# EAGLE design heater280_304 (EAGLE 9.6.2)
DATABASE: Z:\Eigene Dateien\Anwendungsdaten\Eagle\partdb\exp.txt
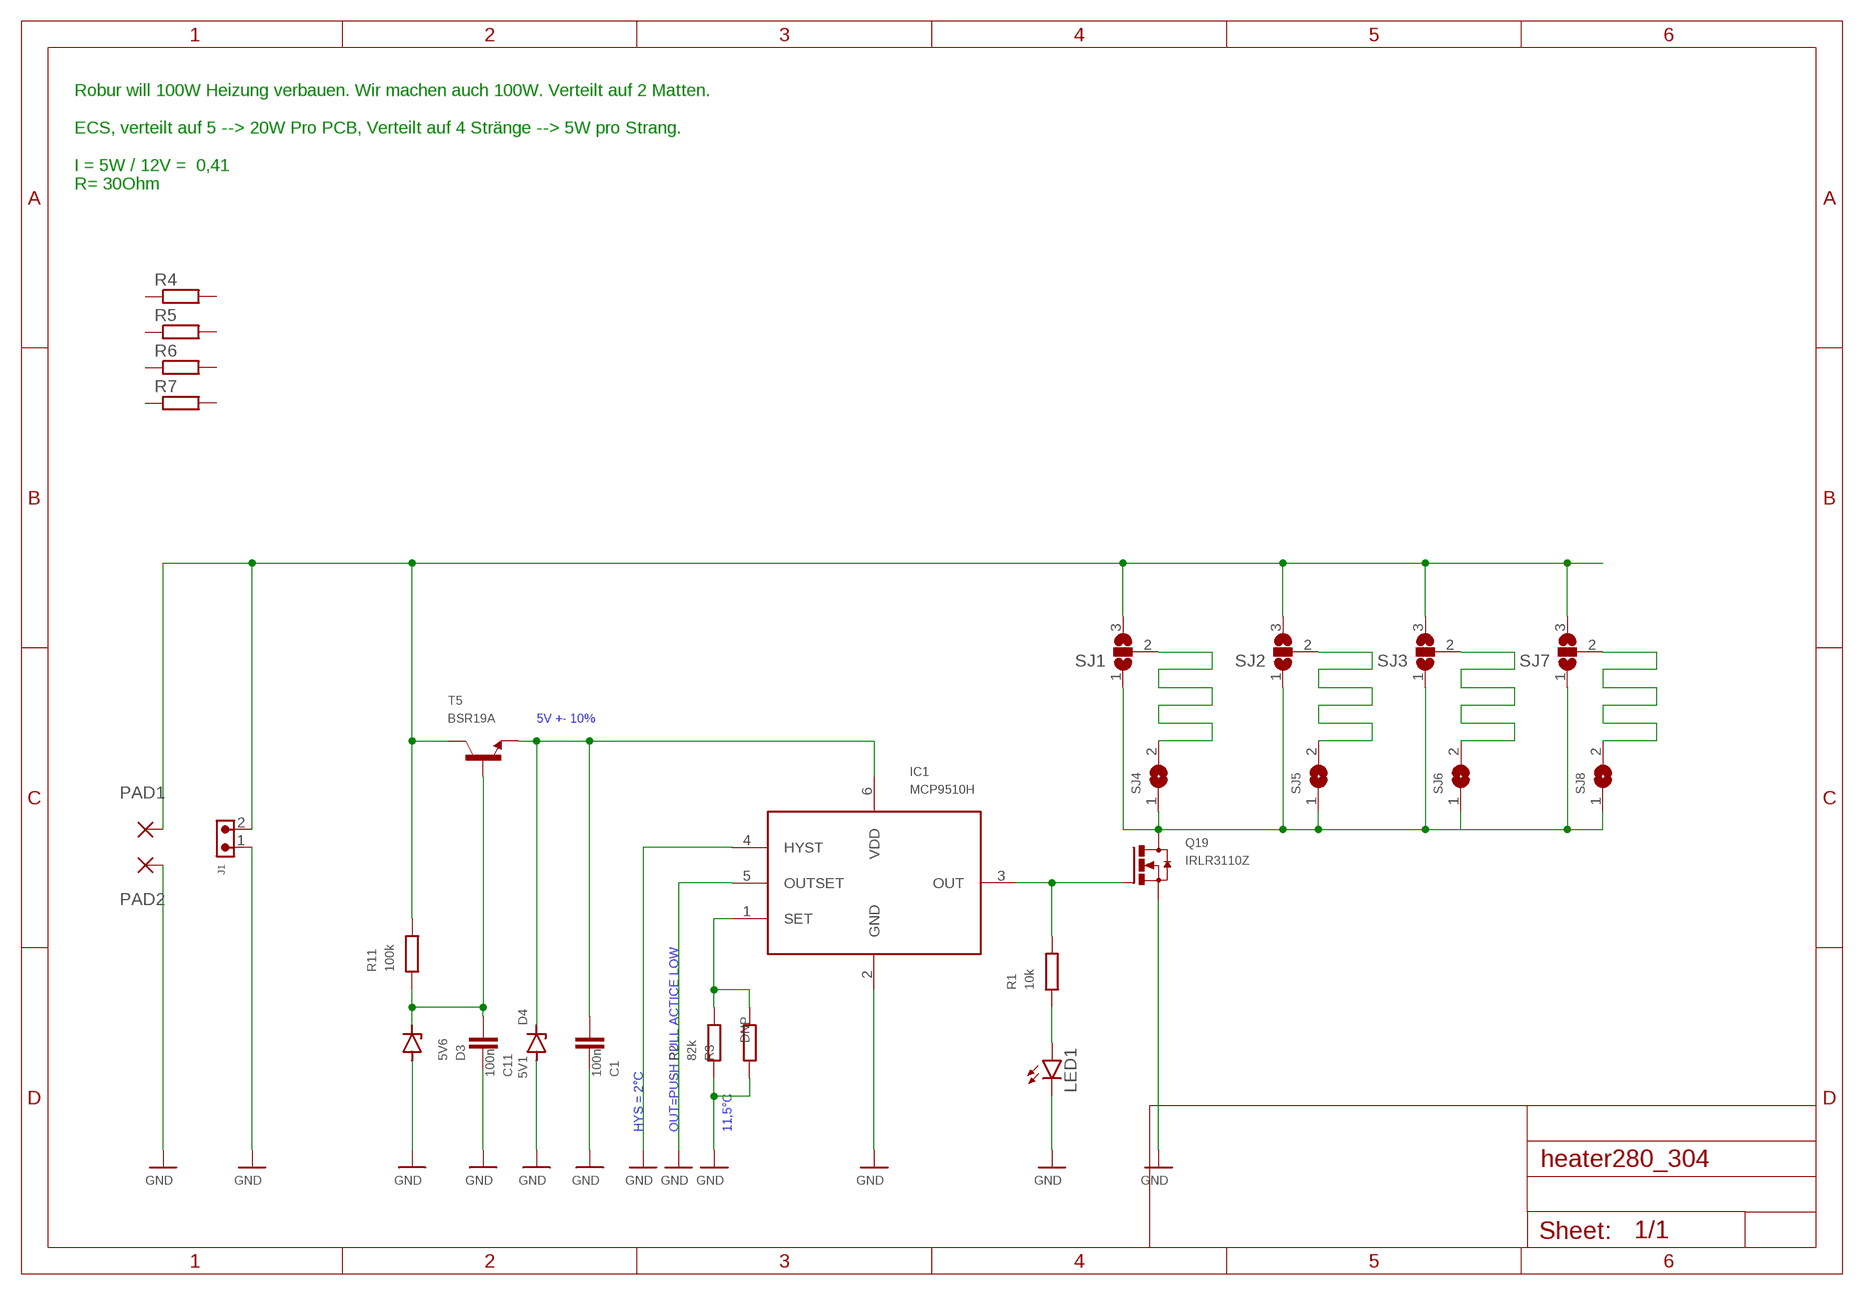
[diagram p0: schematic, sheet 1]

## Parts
C1  100n  C-EUC0603  [C0603]
C11  100n  C-EUC0603  [C0603]
D3  5V6  ZENER-DIODESOD80C  [SOD80C]
D4  5V1  ZENER-DIODESOD80C  [SOD80C]
IC1  MCP9510H  MCP9509  [SOT23-6]
J1  691322110002  [691322110002]
LED1  LEDSML0603  [SML0603]
PAD1  3,81/1,4  [3,81/1,4]
PAD2  3,81/1,4  [3,81/1,4]
Q19  IRLR3110Z  IRFR2607  [D-PACK]
R1  10k  R-EU_R0603  [R0603]
R2  82k  R-EU_R0603  [R0603]
R3  R-EU_R0603  [R0603]
R4  R-EU_R1206  [R1206]
R5  R-EU_R1206  [R1206]
R6  R-EU_R1206  [R1206]
R7  R-EU_R1206  [R1206]
R11  100k  R-EU_R0603  [R0603]
SJ1  SJ2W  [SJ_2]
SJ2  SJ2W  [SJ_2]
SJ3  SJ2W  [SJ_2]
SJ4  SJ  [SJ]
SJ5  SJ  [SJ]
SJ6  SJ  [SJ]
SJ7  SJ2W  [SJ_2]
SJ8  SJ  [SJ]
T5  BSR19A  MMBT2222ALT1-NPN-SOT23-BEC  [SOT23-BEC]

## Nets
+UB: J1.2 PAD1.1(P) R11.2 SJ1.3 SJ2.3 SJ3.3 SJ7.3 T5.C
GND: C1.2 C11.2 D3.A D4.A IC1.2(GND) IC1.4(HYST) IC1.5(OUTSET) J1.1 LED1.C PAD2.1(P) Q19.3(S) R2.1 R3.1
N$1: IC1.3(OUT) Q19.1(G) R1.2
N$2: SJ1.2 SJ4.2
N$3: C11.1 D3.C R11.1 T5.B
N$4: IC1.1(SET) R2.2 R3.2
N$5: C1.1 D4.C IC1.6(VDD) T5.E
N$6: LED1.A R1.1
N$7: SJ2.2 SJ5.2
N$8: SJ3.2 SJ6.2
N$9: SJ7.2 SJ8.2
N$11: Q19.4(D) SJ1.1 SJ2.1 SJ3.1 SJ4.1 SJ5.1 SJ6.1 SJ7.1 SJ8.1
Unconnected: R4.1 R4.2 R5.1 R5.2 R6.1 R6.2 R7.1 R7.2

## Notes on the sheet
- Robur will 100W Heizung verbauen. Wir machen auch 100W. Verteilt auf 2 Matten.
  
  ECS, verteilt auf 5 --> 20W Pro PCB, Verteilt auf 4 Stränge --> 5W pro Strang.
  
  I = 5W / 12V =  0,41
  R= 30Ohm
- 5V +- 10%
- HYS = 2°C | OUT=PUSH PULL ACTICE LOW | 11,5°C

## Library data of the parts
C1 C11 = rcl:C-EU: CAPACITOR, European symbol; PARTNO: C067; SPICEPREFIX: C
D3 = diode:ZENER-DIODE: Z-Diode; PARTNO: D013
D4 = diode:ZENER-DIODE: Z-Diode; PARTNO: D012
IC1 = mcp9509:MCP9509; PARTNO: IC333
J1 = Wurth_Connectors_WR-TBL Pluggable Connector:691322110002: WR-TBL Serie 3221 - 3.50 mm Horizontal PCB Header; DATASHEET-URL: https://www.we-online.com/catalog/datasheet/691322110002.pdf; IR-UL: 10A; IR-VDE: 10.5A; MOUNT: THT; PART-NUMBER: 691322110002; PARTNO: CON212; PINS: 2; PITCH: 3.5mm; TYPE: Horizontal; WORKING-VOLTAGE-UL: 300V (AC); WORKING-VOLTAGE-VDE: 300V (AC)
LED1 = led:LED: LED; PARTNO: D078
PAD1 PAD2 = wirepad:3,81/1,4: THROUGH-HOLE PAD
Q19 = IRFR2607:IRFR2607; PARTNO: T086
R1 = rcl:R-EU_: RESISTOR, European symbol; PARTNO: R221; SPICEPREFIX: R
R2 = rcl:R-EU_: RESISTOR, European symbol; PARTNO: R243; SPICEPREFIX: R
R3 = rcl:R-EU_: RESISTOR, European symbol; DNP: T; PARTNO: R245; SPICEPREFIX: R
R4-R7 = rcl:R-EU_: RESISTOR, European symbol; PARTNO: R493; SPICEPREFIX: R
R11 = rcl:R-EU_: RESISTOR, European symbol; PARTNO: R245; SPICEPREFIX: R
SJ1-SJ3 SJ7 = jumper:SJ2W: SMD solder JUMPER
SJ4-SJ6 SJ8 = jumper:SJ: SMD solder JUMPER
T5 = transistor-neu-to92:*-NPN-: NPN Transistror; PARTNO: T056

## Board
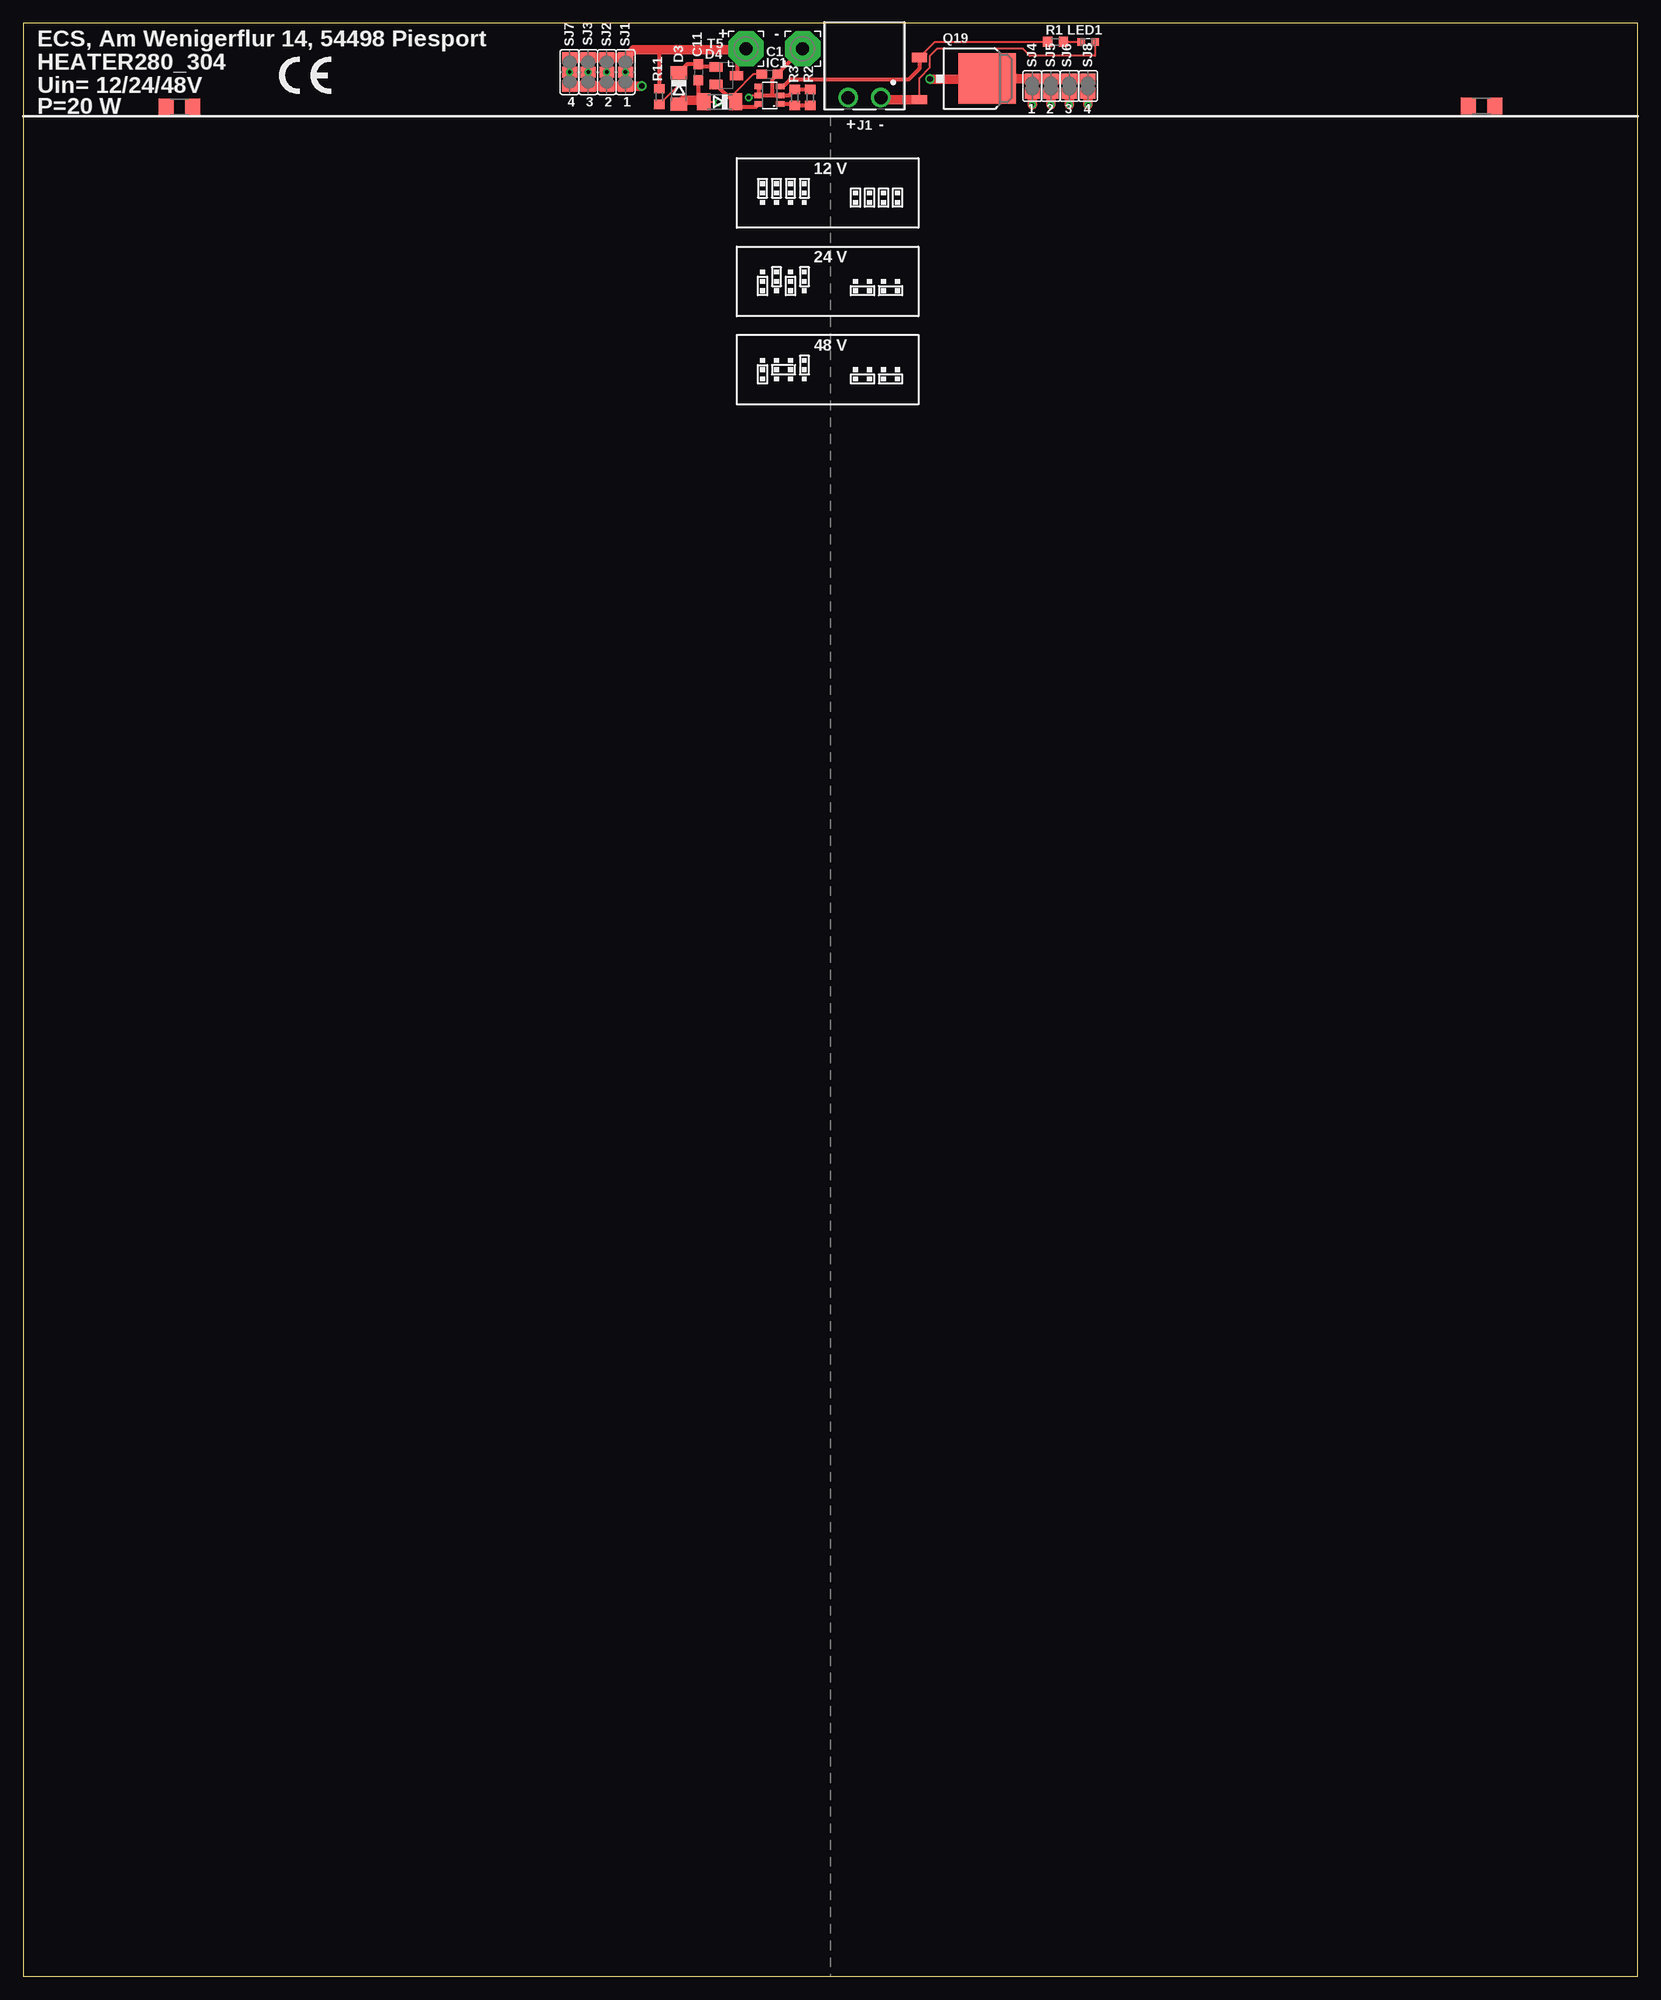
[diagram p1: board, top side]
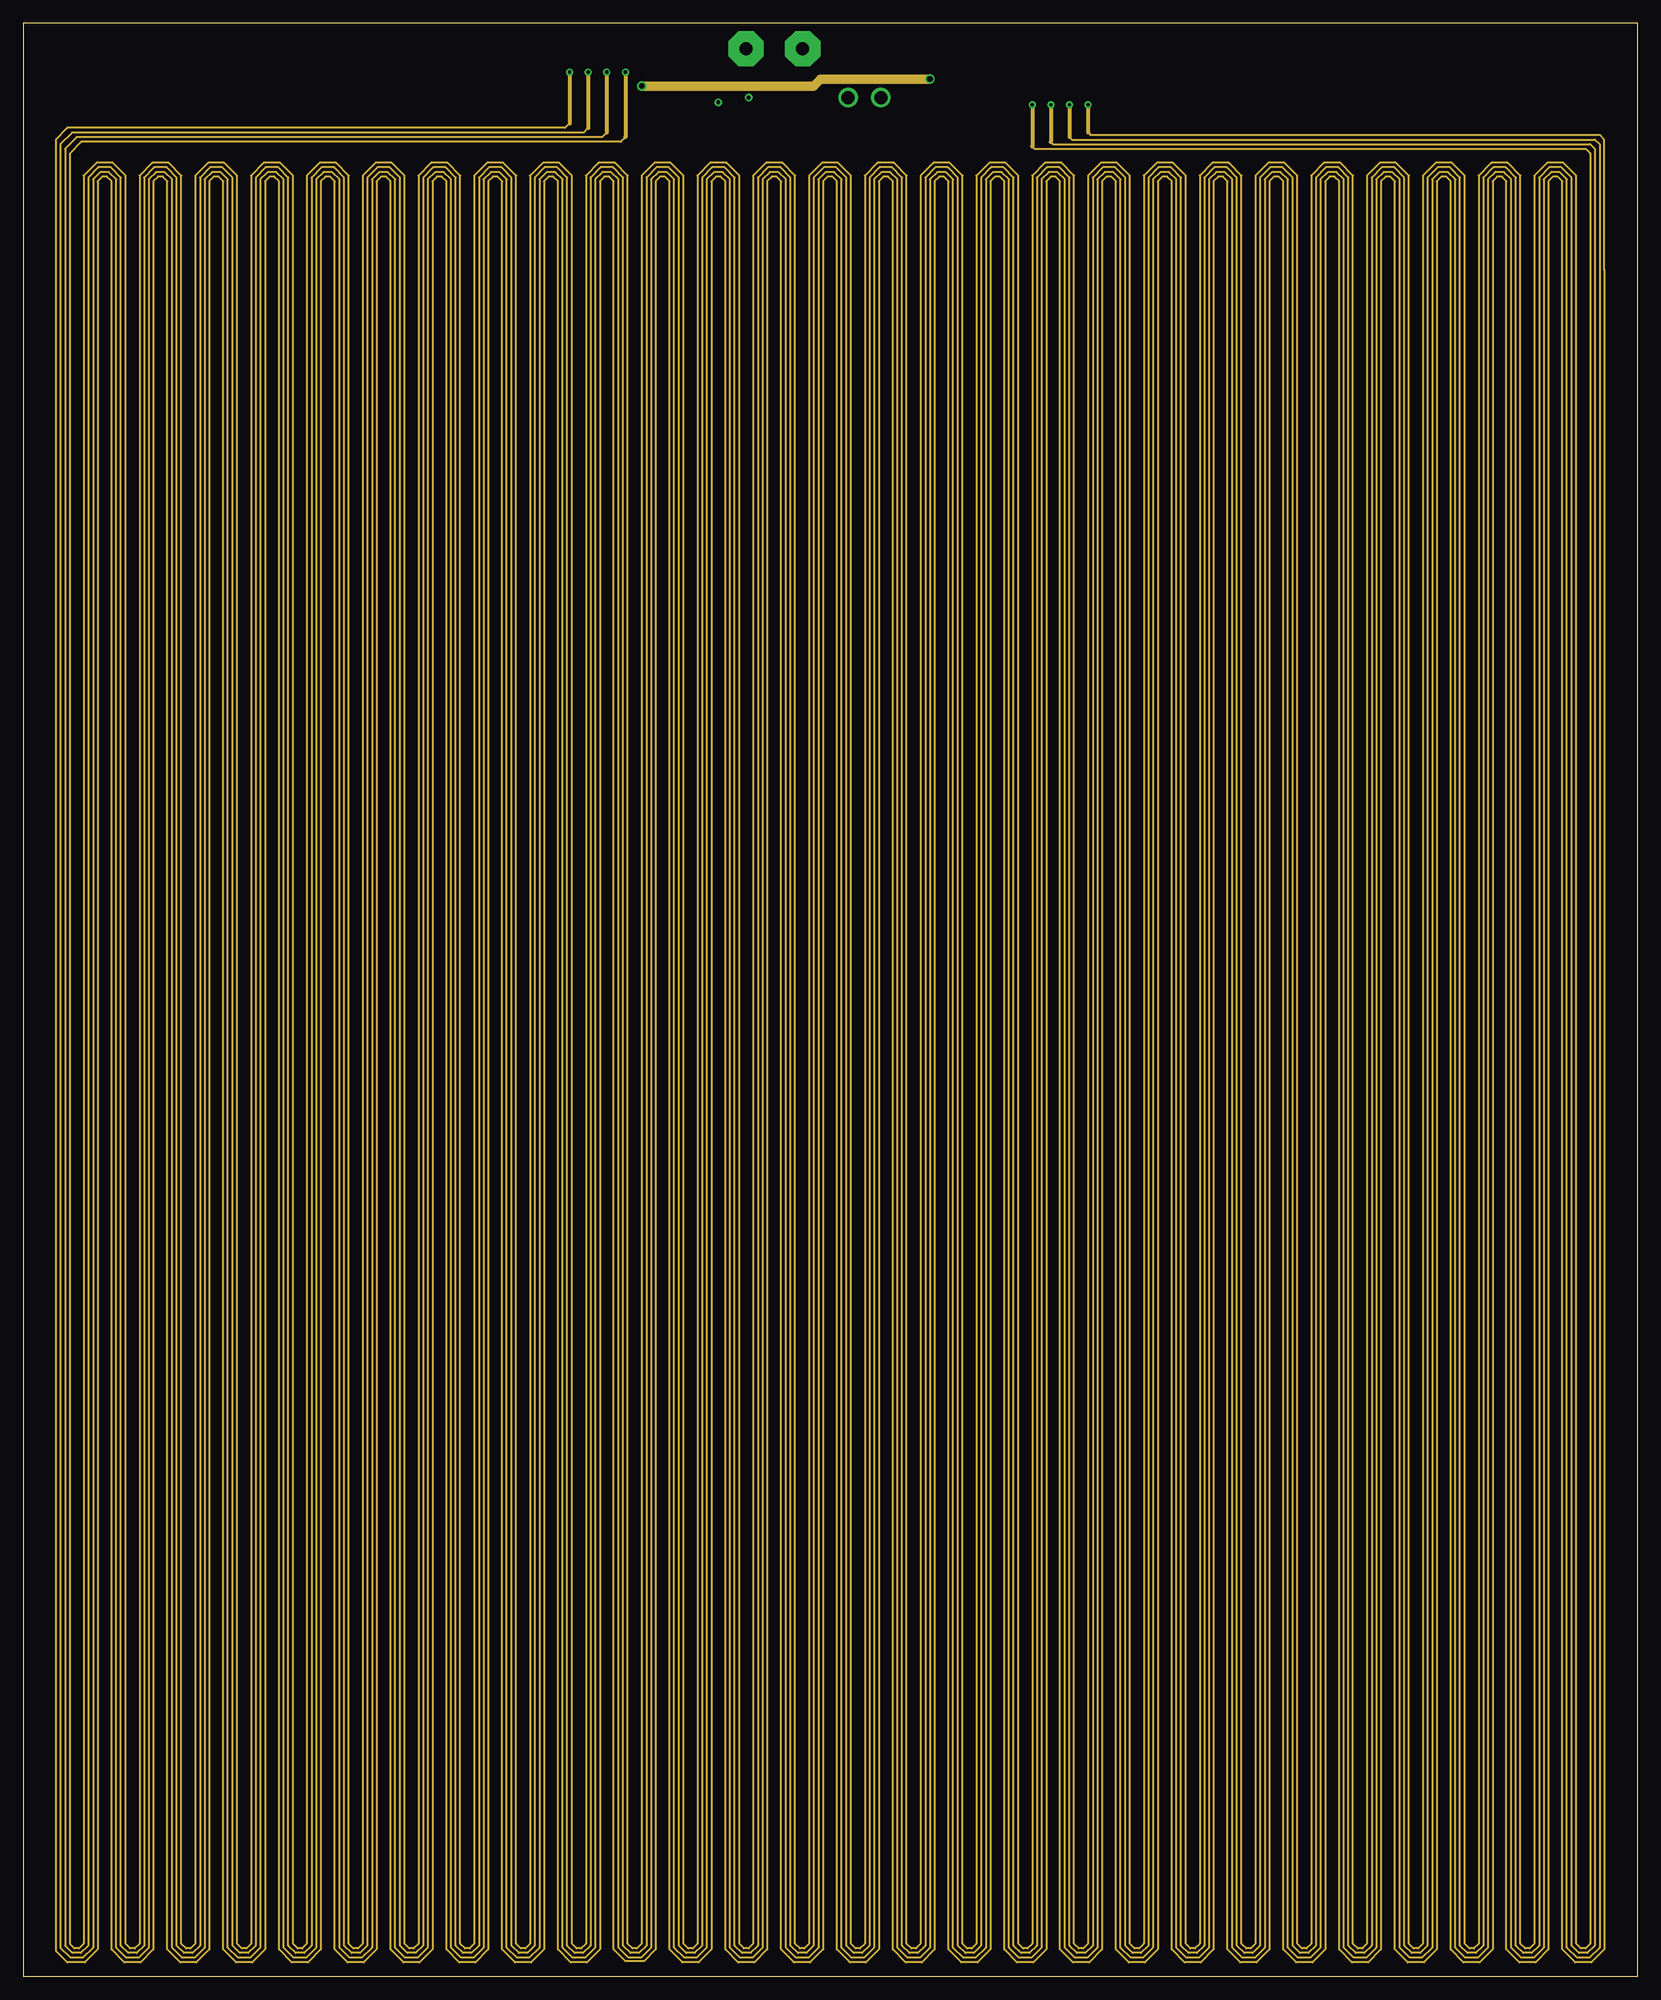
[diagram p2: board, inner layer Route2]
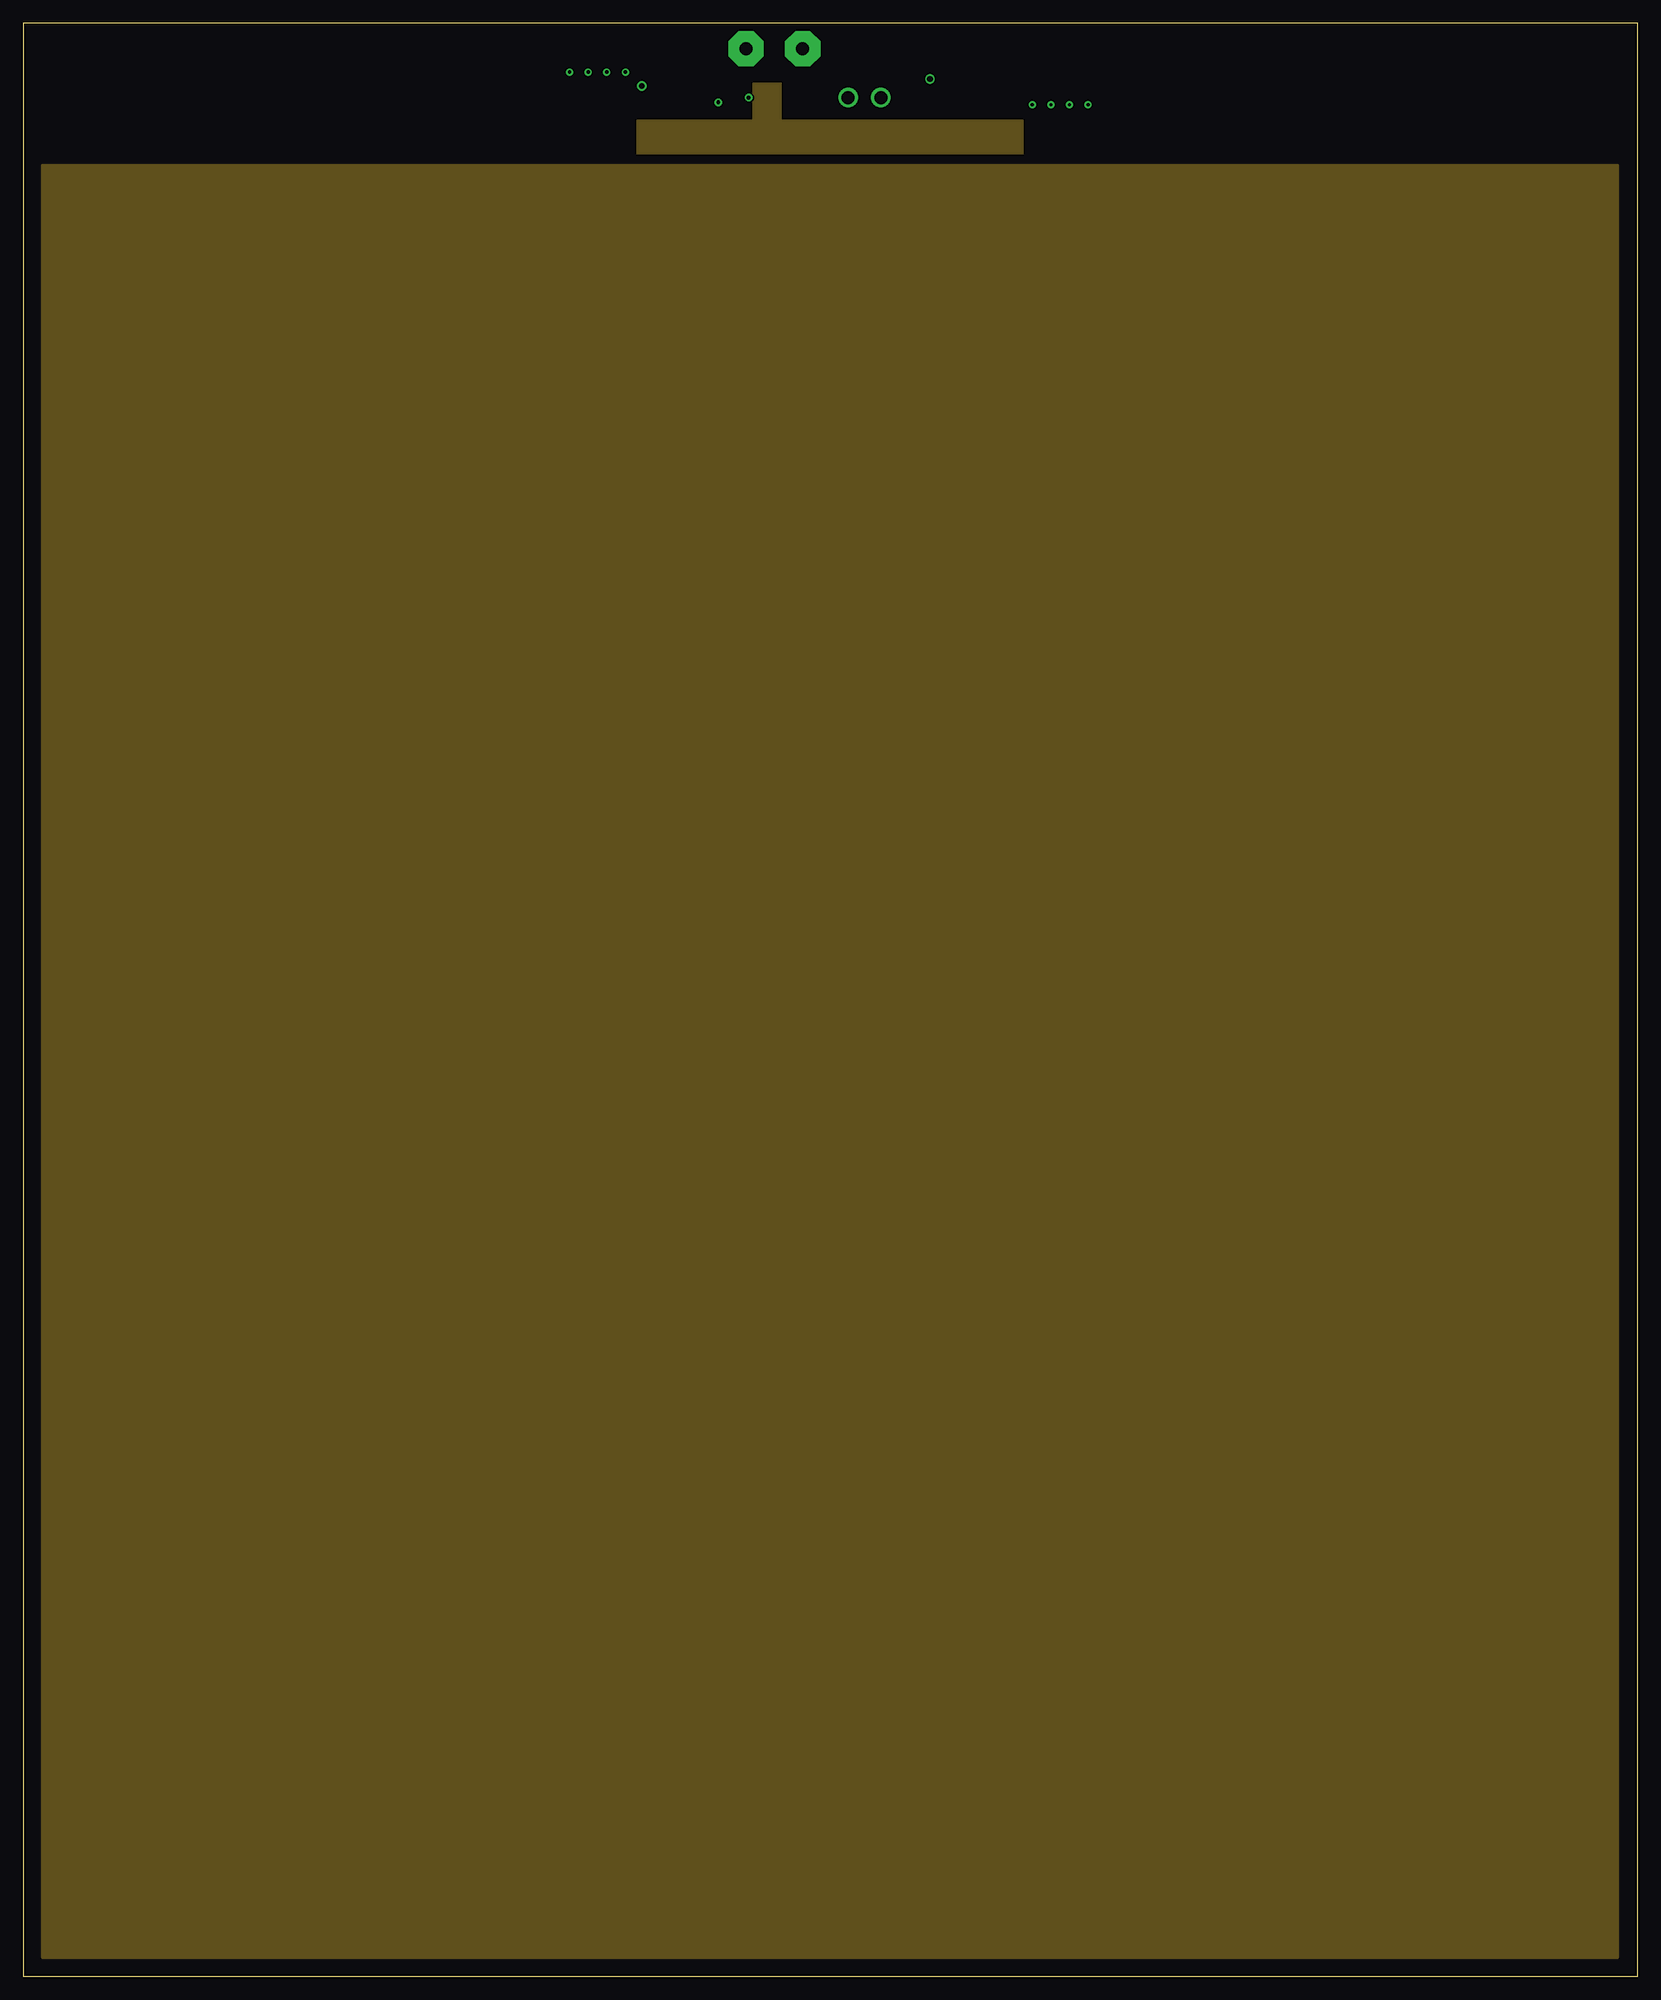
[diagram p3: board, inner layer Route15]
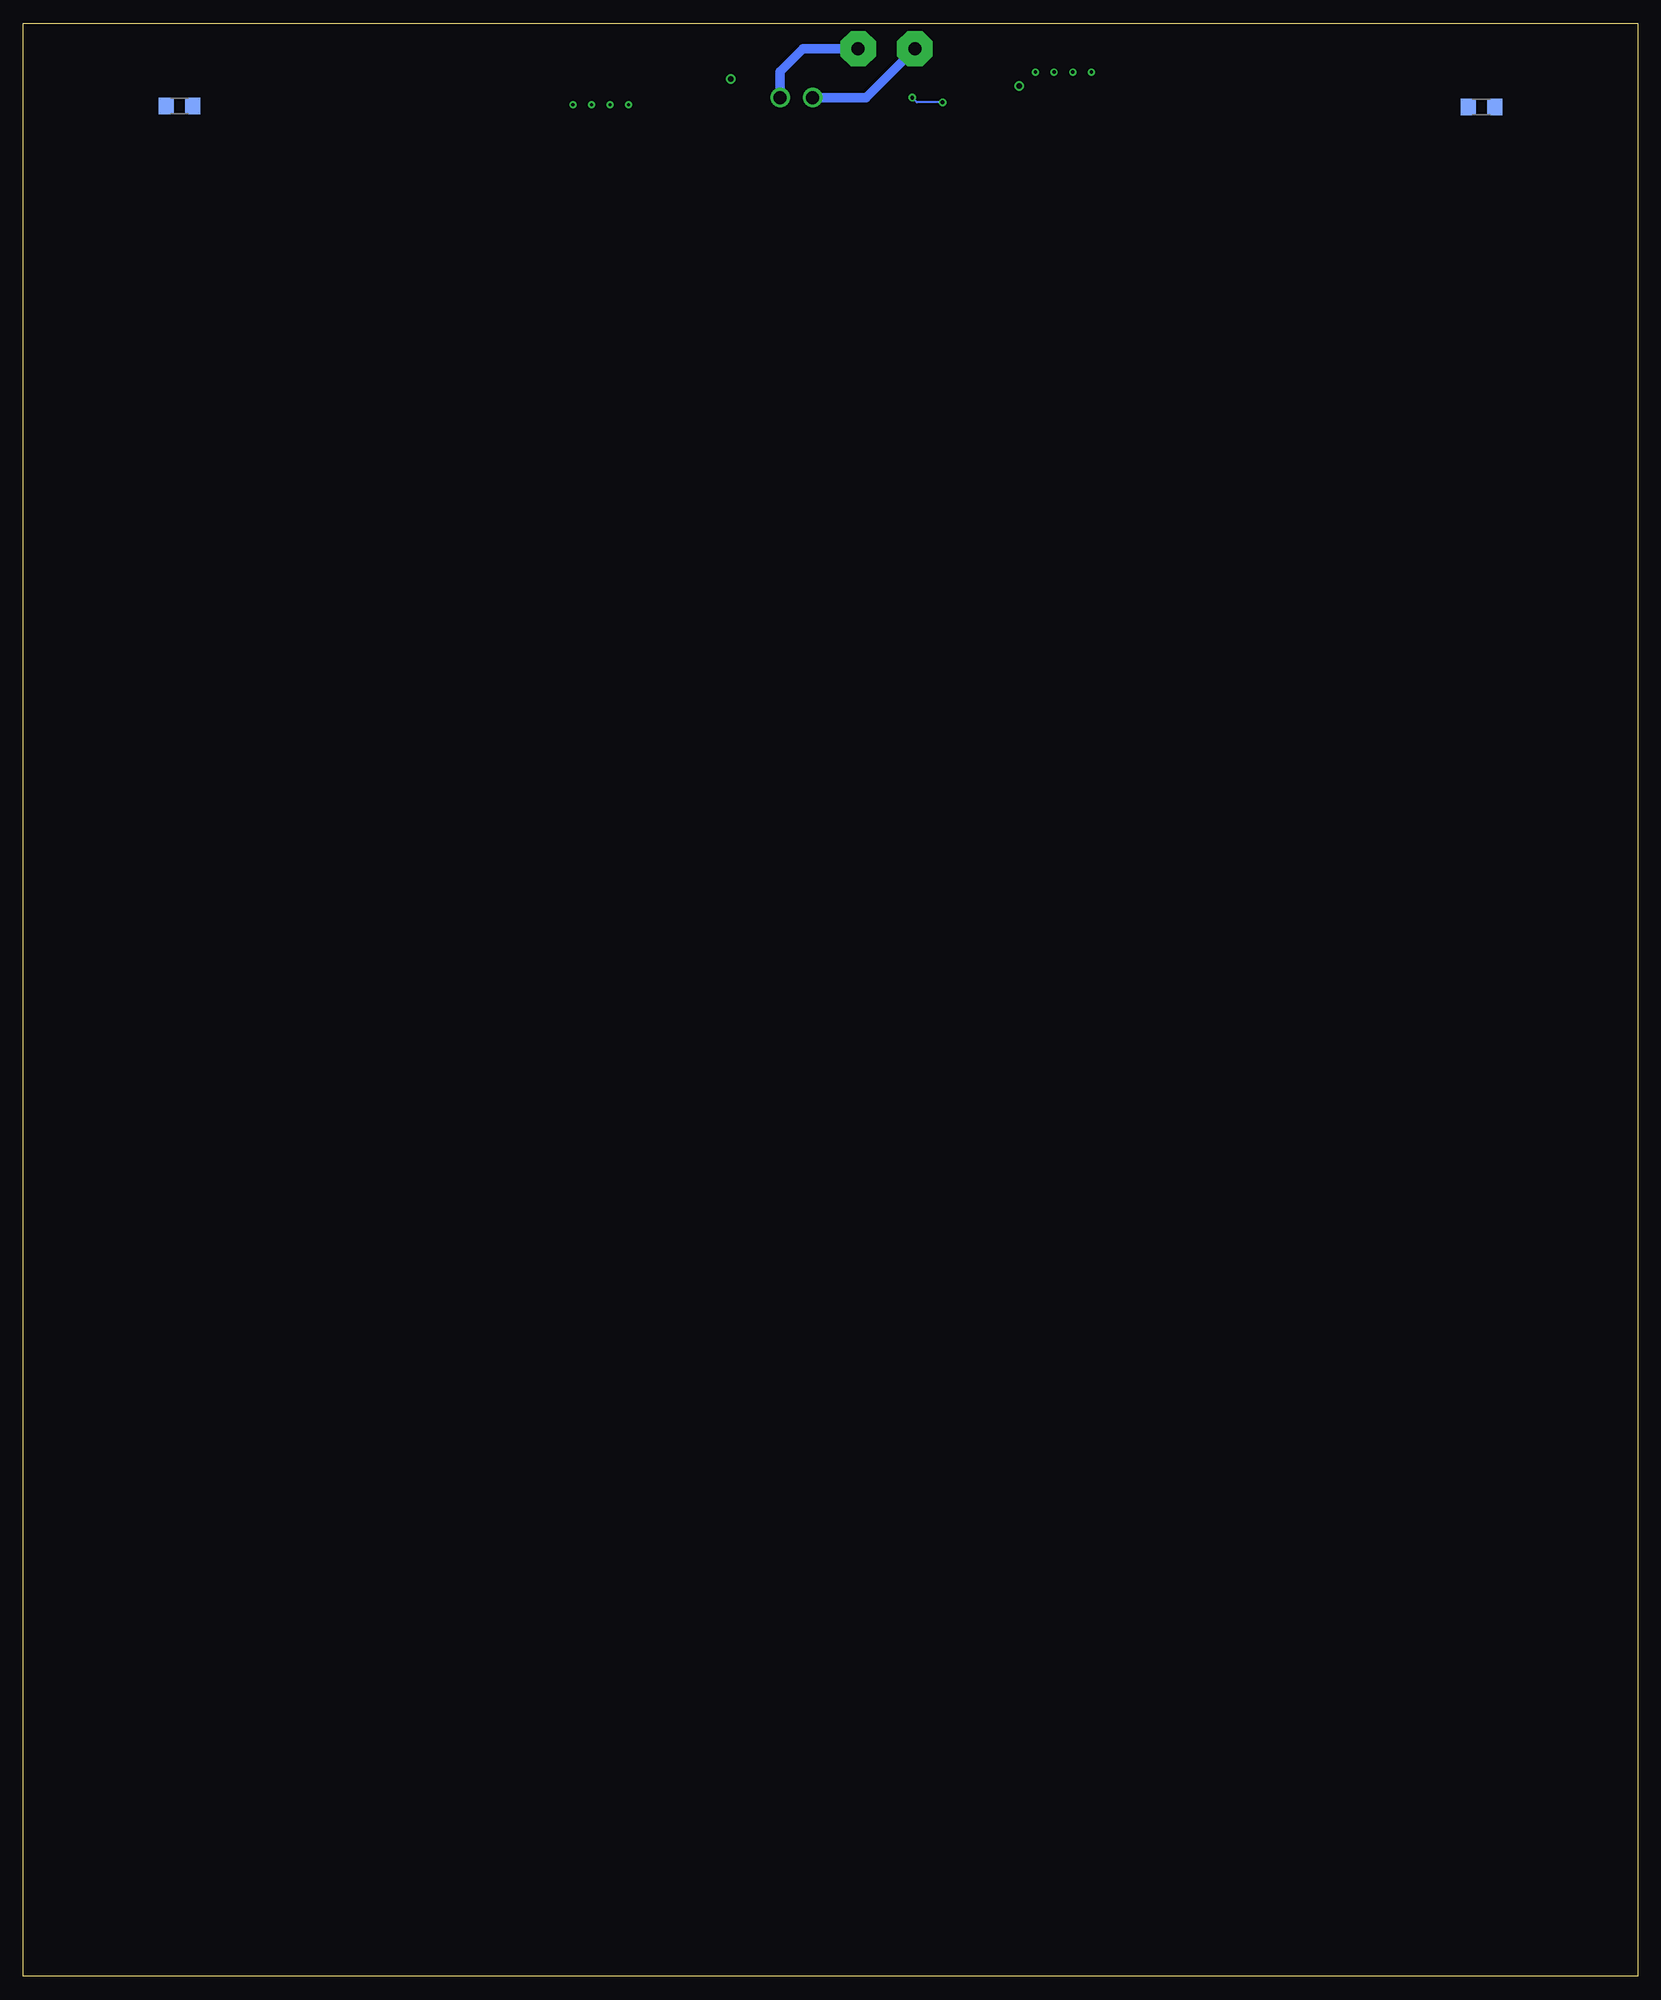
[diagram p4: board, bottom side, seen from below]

Size 173.6 x 210 mm. Coordinates in mm from the lower left corner, seen from the top.
Outline: 0,0 173.6,0 173.6,210 0,210 0,0
Copper layers (1+2*15+16): Top 0.035mm / dielectric 1.5mm / Route2 0.035mm / dielectric 0.15mm / Route15 0.035mm / dielectric 0.2mm / Bottom 0.035mm
Design rules "default *": minimum track width 6mil, minimum drill 0.35mm, track to track 6mil, track to pad 6mil, pad to pad 6mil, via to via 6mil, smd to smd 6mil, copper to edge 40mil, drill to drill 6mil, minimum pad ring 10mil, minimum via ring 8mil, stop-mask expansion 4mil, vias tented up to drill 0mil, thermal gap 10mil

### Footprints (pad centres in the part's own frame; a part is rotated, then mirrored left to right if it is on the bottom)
C0603 = smd 1.1 x 1: 1 -0.85,0; 2 0.85,0
SOD80C = smd 1.4 x 1.8: A 1.7,0; C -1.7,0
SOT23-6 = smd 0.6 x 0.9: 1 -0.95,-1.15; 2 0,-1.15; 3 0.95,-1.15; 4 0.95,1.15; 5 0,1.15; 6 -0.95,1.15
691322110002 = drill 1.4: 1 -1.75,0; 2 1.75,0
SML0603 = smd 0.8 x 0.8: A 0.75,0; C -0.75,0
3,81/1,4 = drill 1.397 pad 3.81 octagon: 1 0,0
D-PACK = smd 1 x 1.6: 1 -2.28,-4.8; 3 2.28,-4.8 | smd 5.4 x 6.2: 4 0,2.5
R0603 = smd 1 x 1.1: 1 -0.85,0; 2 0.85,0
R1206 = smd 1.6 x 1.803: 1 -1.422,0; 2 1.422,0
SJ_2 = smd 1.168 x 1.6: 1 -1.524,0; 2 0,0; 3 1.524,0
SJ = smd 1.168 x 1.6: 1 -0.762,0; 2 0.762,0
SOT23-BEC = smd 1 x 1.4: B -0.95,-1.1; C 0,1.1; E 0.95,-1.1

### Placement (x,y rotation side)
C1  80.27,204.52 0 top
C11  72.6,204.73 270 top
D3  70.5,203 270 top
D4  74.88,201.55 180 top
IC1  80.25,202.25 90 top
J1  90.46,202.01 180 top
LED1  114.5,208 180 top
PAD1  77.72,207.26 0 top
PAD2  83.82,207.26 0 top
Q19  101.16,204.05 270 top
R1  111,208 180 top
R2  84.64,202.02 270 top
R3  82.97,202.02 270 top
R4  16.8,201 180 top
R5  16.8,201 0 bottom
R6  156.8,201.1 0 top
R7  156.8,201.1 0 bottom
R11  68.4,202.12 90 top
SJ1  64.75,204.75 90 top
SJ2  62.75,204.75 90 top
SJ3  60.75,204.75 90 top
SJ4  108.5,203.25 270 top
SJ5  110.5,203.25 270 top
SJ6  112.5,203.25 270 top
SJ7  58.75,204.75 90 top
SJ8  114.5,203.25 270 top
T5  75.61,204.36 270 top
U$1  [CE-4MM]  27.5,202.38 0 top

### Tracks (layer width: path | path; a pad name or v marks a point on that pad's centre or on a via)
+UB
  Top 0.406: T5.C 76.75,204.4 76.75,206.29 77.61,207.15 PAD1.1 | R11.2 68.4,207.04 68.5,207.15
  Top 1.016: SJ7.3 SJ3.3 SJ2.3 SJ1.3 65.62,207.15 68.5,207.15 77.61,207.15
  Bottom 1.016: PAD1.1 82.97,202.01 J1.2
GND  (via drill 0.4)
  Top 0.2: LED1.C 115.25,206.5 108.25,206.5 107.5,207.25 98.25,207.25 97.5,206.5 97.5,205.25 96.36,204.11 Q19.3 | D4.A 74.7,201.55 v74.75,201.5 | v78,202 78.25,202.25 IC1.5
  Top 0.406: D4.A 72.6,202.13 C11.2 | 80.56,202.25 IC1.2 82.35,202.25 R3.1 R2.1 | 80.56,202.25 80.56,203.96 C1.2 81.12,204.56 PAD2.1 | IC1.4 IC1.5 80.56,202.25
  Top 1.016: D3.A 70.95,201.75 72.98,201.75 D4.A | Q19.3 92.45,201.77 J1.1
  Bottom 0.2: v74.75,201.5 77.5,201.5 v78,202
  Bottom 1.016: J1.1 92.21,204.79 89.74,207.26 PAD2.1
N$1
  Top 0.2: Q19.1 98.03,208 R1.2
  Top 0.406: IC1.3 81.7,203.2 82.5,204 95.25,204 96.36,205.11 Q19.1
N$2  (via drill 0.35, 0.35 pad 0.21)
  Top 1.016: SJ4.2 v108.5,201.25
  Route2 0.2: 108.5,196.75 108.75,196.5 168,196.5 168.5,196 168.5,3.5 168,3 167.5,3 167,3.5 167,193.62 165.62,195 163.88,195 162.5,193.62 162.5,3.5 162,3 161.5,3 161,3.5 161,193.62 159.62,195 157.88,195 156.5,193.62 156.5,3.5 156,3 155.5,3 155,3.5 155,193.62 153.62,195 151.88,195 150.5,193.62 150.5,3.5 150,3 149.5,3 149,3.5 149,193.62 147.62,195 145.88,195 144.5,193.62 144.5,3.5 144,3 143.5,3 143,3.5 143,193.62 141.62,195 139.88,195 138.5,193.62 138.5,3.5 138,3 137.5,3 137,3.5 137,193.62 135.62,195 133.88,195 132.5,193.62 132.5,3.5 132,3 131.5,3 131,3.5 131,193.62 129.62,195 127.88,195 126.5,193.62 126.5,3.5 126,3 125.5,3 125,3.5 125,193.62 123.62,195 121.88,195 120.5,193.62 120.5,3.5 120,3 119.5,3 119,3.5 119,193.62 117.62,195 115.88,195 114.5,193.62 114.5,3.5 114,3 113.5,3 113,3.5 113,193.62 111.62,195 109.88,195 108.5,193.62 108.5,3.5 108,3 107.5,3 107,3.5 107,193.62 105.62,195 103.88,195 102.5,193.62 102.5,3.5 102,3 101.5,3 101,3.5 101,193.62 99.62,195 97.88,195 96.5,193.62 96.5,3.5 96,3 95.5,3 95,3.5 95,193.62 93.62,195 91.88,195 90.5,193.62 90.5,3.5 90,3 89.5,3 89,3.5 89,193.62 87.62,195 85.88,195 84.5,193.62 84.5,3.5 84,3 83.5,3 83,3.5 83,193.62 81.62,195 79.88,195 78.5,193.62 78.5,3.5 78,3 77.5,3 77,3.5 77,193.62 75.62,195 73.88,195 72.5,193.62 72.5,3.5 72,3 71.5,3 71,3.5 71,193.62 69.62,195 67.88,195 66.5,193.62 66.5,3.5 66,3 65.5,3 65,3.5 65,193.62 63.62,195 61.88,195 60.5,193.62 60.5,3.5 60,3 59.5,3 59,3.5 59,193.62 57.62,195 55.88,195 54.5,193.62 54.5,3.5 54,3 53.5,3 53,3.5 53,193.62 51.62,195 49.88,195 48.5,193.62 48.5,3.5 48,3 47.5,3 47,3.5 47,193.62 45.62,195 43.88,195 42.5,193.62 42.5,3.5 42,3 41.5,3 41,3.5 41,193.62 39.62,195 37.88,195 36.5,193.62 36.5,3.5 36,3 35.5,3 35,3.5 35,193.62 33.62,195 31.88,195 30.5,193.62 30.5,3.5 30,3 29.5,3 29,3.5 29,193.62 27.62,195 25.88,195 24.5,193.62 24.5,3.5 24,3 23.5,3 23,3.5 23,193.62 21.62,195 19.88,195 18.5,193.62 18.5,3.5 18,3 17.5,3 17,3.5 17,193.62 15.62,195 13.88,195 12.5,193.62 12.5,3.5 12,3 11.5,3 11,3.5 11,193.62 9.62,195 7.88,195 6.5,193.62 6.5,3.5 6,3 5.5,3 5,3.5 5,196 6.26,197.25 64.25,197.25 64.75,197.75
  Route2 0.406: v108.5,201.25 108.5,196.75 | SJ1.2 64.75,197.75
  other vias: 64.75,204.75
N$3
  Top 0.2: R11.1 70.5,203.37 D3.C
  Top 0.406: D3.C 71.38,205.58 C11.1 72.87,205.31 T5.B
N$4
  Top 0.406: IC1.1 82.97,201.3 R3.2 R2.2
N$5
  Top 0.2: C1.1 79.4,204.5 78.5,204.5 76.58,202.58 D4.C
  Top 0.406: T5.E 76.37,201.55 D4.C 76.83,201.3 76.95,201.3 77.25,201 78.77,201 IC1.6
N$6
  Top 0.2: R1.1 LED1.A
N$7  (via drill 0.35, 0.35 pad 0.21)
  Top 1.016: SJ5.2 v110.5,201.25
  Route2 0.2: 110.5,197.25 110.75,197 168.5,197 169,196.5 169,3.29 168.21,2.5 167.29,2.5 166.5,3.29 166.5,193.41 165.41,194.5 164.09,194.5 163,193.41 163,3.29 162.21,2.5 161.29,2.5 160.5,3.29 160.5,193.41 159.41,194.5 158.09,194.5 157,193.41 157,3.29 156.21,2.5 155.29,2.5 154.5,3.29 154.5,193.41 153.41,194.5 152.09,194.5 151,193.41 151,3.29 150.21,2.5 149.29,2.5 148.5,3.29 148.5,193.41 147.41,194.5 146.09,194.5 145,193.41 145,3.29 144.21,2.5 143.29,2.5 142.5,3.29 142.5,193.41 141.41,194.5 140.09,194.5 139,193.41 139,3.29 138.21,2.5 137.29,2.5 136.5,3.29 136.5,193.41 135.41,194.5 134.09,194.5 133,193.41 133,3.29 132.21,2.5 131.29,2.5 130.5,3.29 130.5,193.41 129.41,194.5 128.09,194.5 127,193.41 127,3.29 126.21,2.5 125.29,2.5 124.5,3.29 124.5,193.41 123.41,194.5 122.09,194.5 121,193.41 121,3.29 120.21,2.5 119.29,2.5 118.5,3.29 118.5,193.41 117.41,194.5 116.09,194.5 115,193.41 115,3.29 114.21,2.5 113.29,2.5 112.5,3.29 112.5,193.41 111.41,194.5 110.09,194.5 109,193.41 109,3.29 108.21,2.5 107.29,2.5 106.5,3.29 106.5,193.41 105.41,194.5 104.09,194.5 103,193.41 103,3.29 102.21,2.5 101.29,2.5 100.5,3.29 100.5,193.41 99.41,194.5 98.09,194.5 97,193.41 97,3.29 96.21,2.5 95.29,2.5 94.5,3.29 94.5,193.41 93.41,194.5 92.09,194.5 91,193.41 91,3.29 90.21,2.5 89.29,2.5 88.5,3.29 88.5,193.41 87.41,194.5 86.09,194.5 85,193.41 85,3.29 84.21,2.5 83.29,2.5 82.5,3.29 82.5,193.41 81.41,194.5 80.09,194.5 79,193.41 79,3.29 78.21,2.5 77.29,2.5 76.5,3.29 76.5,193.41 75.41,194.5 74.09,194.5 73,193.41 73,3.29 72.21,2.5 71.29,2.5 70.5,3.29 70.5,193.41 69.41,194.5 68.09,194.5 67,193.41 67,3.29 66.21,2.5 65.29,2.5 64.5,3.29 64.5,193.41 63.41,194.5 62.09,194.5 61,193.41 61,3.29 60.21,2.5 59.29,2.5 58.5,3.29 58.5,193.41 57.41,194.5 56.09,194.5 55,193.41 55,3.29 54.21,2.5 53.29,2.5 52.5,3.29 52.5,193.41 51.41,194.5 50.09,194.5 49,193.41 49,3.29 48.21,2.5 47.29,2.5 46.5,3.29 46.5,193.41 45.41,194.5 44.09,194.5 43,193.41 43,3.29 42.21,2.5 41.29,2.5 40.5,3.29 40.5,193.41 39.41,194.5 38.09,194.5 37,193.41 37,3.29 36.21,2.5 35.29,2.5 34.5,3.29 34.5,193.41 33.41,194.5 32.09,194.5 31,193.41 31,3.29 30.21,2.5 29.29,2.5 28.5,3.29 28.5,193.41 27.41,194.5 26.09,194.5 25,193.41 25,3.29 24.21,2.5 23.29,2.5 22.5,3.29 22.5,193.41 21.41,194.5 20.09,194.5 19,193.41 19,3.29 18.21,2.5 17.29,2.5 16.5,3.29 16.5,193.41 15.41,194.5 14.09,194.5 13,193.41 13,3.29 12.21,2.5 11.29,2.5 10.5,3.29 10.5,193.41 9.41,194.5 8.09,194.5 7,193.41 7,3.29 6.21,2.5 5.29,2.5 4.5,3.29 4.5,196.5 5.75,197.75 62.25,197.75 62.75,198.25
  Route2 0.406: v110.5,201.25 110.5,197.25 | SJ2.2 62.75,198.25
  other vias: 62.75,204.75
N$8  (via drill 0.35, 0.35 pad 0.21)
  Top 1.016: SJ6.2 v112.5,201.25
  Route2 0.2: 112.5,197.75 112.75,197.5 169,197.5 169.5,197 169.5,3.09 168.41,2 167.09,2 166,3.09 166,193.21 165.21,194 164.29,194 163.5,193.21 163.5,3.09 162.41,2 161.09,2 160,3.09 160,193.21 159.21,194 158.29,194 157.5,193.21 157.5,3.09 156.41,2 155.09,2 154,3.09 154,193.21 153.21,194 152.29,194 151.5,193.21 151.5,3.09 150.41,2 149.09,2 148,3.09 148,193.21 147.21,194 146.29,194 145.5,193.21 145.5,3.09 144.41,2 143.09,2 142,3.09 142,193.21 141.21,194 140.29,194 139.5,193.21 139.5,3.09 138.41,2 137.09,2 136,3.09 136,193.21 135.21,194 134.29,194 133.5,193.21 133.5,3.09 132.41,2 131.09,2 130,3.09 130,193.21 129.21,194 128.29,194 127.5,193.21 127.5,3.09 126.41,2 125.09,2 124,3.09 124,193.21 123.21,194 122.29,194 121.5,193.21 121.5,3.09 120.41,2 119.09,2 118,3.09 118,193.21 117.21,194 116.29,194 115.5,193.21 115.5,3.09 114.41,2 113.09,2 112,3.09 112,193.21 111.21,194 110.29,194 109.5,193.21 109.5,3.09 108.41,2 107.09,2 106,3.09 106,193.21 105.21,194 104.29,194 103.5,193.21 103.5,3.09 102.41,2 101.09,2 100,3.09 100,193.21 99.21,194 98.29,194 97.5,193.21 97.5,3.09 96.41,2 95.09,2 94,3.09 94,193.21 93.21,194 92.29,194 91.5,193.21 91.5,3.09 90.41,2 89.09,2 88,3.09 88,193.21 87.21,194 86.29,194 85.5,193.21 85.5,3.09 84.41,2 83.09,2 82,3.09 82,193.21 81.21,194 80.29,194 79.5,193.21 79.5,3.09 78.41,2 77.09,2 76,3.09 76,193.21 75.21,194 74.29,194 73.5,193.21 73.5,3.09 72.41,2 71.09,2 70,3.09 70,193.21 69.21,194 68.29,194 67.5,193.21 67.5,3.09 66.41,2 65.09,2 64,3.09 64,193.21 63.21,194 62.29,194 61.5,193.21 61.5,3.09 60.41,2 59.09,2 58,3.09 58,193.21 57.21,194 56.29,194 55.5,193.21 55.5,3.09 54.41,2 53.09,2 52,3.09 52,193.21 51.21,194 50.29,194 49.5,193.21 49.5,3.09 48.41,2 47.09,2 46,3.09 46,193.21 45.21,194 44.29,194 43.5,193.21 43.5,3.09 42.41,2 41.09,2 40,3.09 40,193.21 39.21,194 38.29,194 37.5,193.21 37.5,3.09 36.41,2 35.09,2 34,3.09 34,193.21 33.21,194 32.29,194 31.5,193.21 31.5,3.09 30.41,2 29.09,2 28,3.09 28,193.21 27.21,194 26.29,194 25.5,193.21 25.5,3.09 24.41,2 23.09,2 22,3.09 22,193.21 21.21,194 20.29,194 19.5,193.21 19.5,3.09 18.41,2 17.09,2 16,3.09 16,193.21 15.21,194 14.29,194 13.5,193.21 13.5,3.09 12.41,2 11.09,2 10,3.09 10,193.21 9.21,194 8.29,194 7.5,193.21 7.5,3.09 6.41,2 5.09,2 4,3.09 4,197 5.25,198.25 60.25,198.25 60.75,198.75
  Route2 0.406: v112.5,201.25 112.5,197.75 | SJ3.2 60.75,198.75
  other vias: 60.75,204.75
N$9  (via drill 0.35, 0.35 pad 0.21)
  Top 1.016: SJ8.2 v114.5,201.25
  Route2 0.2: 114.5,198.25 114.75,198 169.5,198 170,197.5 170,183.48 | 170,183.48 | 170,183.48 170,2.88 168.62,1.5 166.88,1.5 165.5,2.88 165.5,193 165,193.5 164.5,193.5 164,193 164,2.88 162.62,1.5 160.88,1.5 159.5,2.88 159.5,193 159,193.5 158.5,193.5 158,193 158,2.88 156.62,1.5 154.88,1.5 153.5,2.88 153.5,193 153,193.5 152.5,193.5 152,193 152,2.88 150.62,1.5 148.88,1.5 147.5,2.88 147.5,193 147,193.5 146.5,193.5 146,193 146,2.88 144.62,1.5 142.88,1.5 141.5,2.88 141.5,193 141,193.5 140.5,193.5 140,193 140,2.88 138.62,1.5 136.88,1.5 135.5,2.88 135.5,193 135,193.5 134.5,193.5 134,193 134,2.88 132.62,1.5 130.88,1.5 129.5,2.88 129.5,193 129,193.5 128.5,193.5 128,193 128,2.88 126.62,1.5 124.88,1.5 123.5,2.88 123.5,193 123,193.5 122.5,193.5 122,193 122,2.88 120.62,1.5 118.88,1.5 117.5,2.88 117.5,193 117,193.5 116.5,193.5 116,193 116,2.88 114.62,1.5 112.88,1.5 111.5,2.88 111.5,193 111,193.5 110.5,193.5 110,193 110,2.88 108.62,1.5 106.88,1.5 105.5,2.88 105.5,193 105,193.5 104.5,193.5 104,193 104,2.88 102.62,1.5 100.88,1.5 99.5,2.88 99.5,193 99,193.5 98.5,193.5 98,193 98,2.88 96.62,1.5 94.88,1.5 93.5,2.88 93.5,193 93,193.5 92.5,193.5 92,193 92,2.88 90.62,1.5 88.88,1.5 87.5,2.88 87.5,193 87,193.5 86.5,193.5 86,193 86,2.88 84.62,1.5 82.88,1.5 81.5,2.88 81.5,193 81,193.5 80.5,193.5 80,193 80,2.88 78.62,1.5 76.88,1.5 75.5,2.88 75.5,193 75,193.5 74.5,193.5 74,193 74,2.88 72.62,1.5 70.88,1.5 69.5,2.88 69.5,193 69,193.5 68.5,193.5 68,193 68,2.88 66.74,1.62 64.76,1.62 63.5,2.88 63.5,193 63,193.5 62.5,193.5 62,193 62,2.88 60.62,1.5 58.88,1.5 57.5,2.88 57.5,193 57,193.5 56.5,193.5 56,193 56,2.88 54.62,1.5 52.88,1.5 51.5,2.88 51.5,193 51,193.5 50.5,193.5 50,193 50,2.88 48.62,1.5 46.88,1.5 45.5,2.88 45.5,193 45,193.5 44.5,193.5 44,193 44,2.88 42.62,1.5 40.88,1.5 39.5,2.88 39.5,193 39,193.5 38.5,193.5 38,193 38,2.88 36.62,1.5 34.88,1.5 33.5,2.88 33.5,193 33,193.5 32.5,193.5 32,193 32,2.88 30.62,1.5 28.88,1.5 27.5,2.88 27.5,193 27,193.5 26.5,193.5 26,193 26,2.88 24.62,1.5 22.88,1.5 21.5,2.88 21.5,193 21,193.5 20.5,193.5 20,193 20,2.88 18.62,1.5 16.88,1.5 15.5,2.88 15.5,193 15,193.5 14.5,193.5 14,193 14,2.88 12.62,1.5 10.88,1.5 9.5,2.88 9.5,193 9,193.5 8.5,193.5 8,193 8,2.88 6.62,1.5 4.75,1.5 3.5,2.75 3.5,197.5 4.75,198.75 58.25,198.75 58.75,199.25
  Route2 0.406: v114.5,201.25 114.5,198.25 | SJ7.2 58.75,199.25
  other vias: 58.75,204.75
N$10
  pour Route15: 78.5,203.5 78.5,199.5 66,199.5 66,196 107.5,196 107.5,199.5 105.5,199.5 81.5,199.5 81.5,203.5
N$11  (via drill 0.6)
  Top 1.016: SJ7.1 SJ3.1 SJ2.1 SJ1.1 66.48,203.23 v66.5,203.25 | SJ8.1 SJ6.1 SJ5.1 SJ4.1 104.65,204.01 103.66,205 Q19.4 103.61,204 v97.5,204
  Route2 1.016: v66.5,203.25 85,203.25 85.75,204 v97.5,204
N$12
  pour Route15: 66,194.75 2,194.75 2,194.5 2,2 171.5,2 171.5,194.75

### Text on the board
tPlace: ECS, Am Wenigerflur 14, 54498 Piesport | + | - | HEATER280_304 | Uin= 12/24/48V | 4 | 3 | 2 | 1 | P=20 W | 1 | 2 | 3 | 4 | + | - | 12 V | 24 V | 48 V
